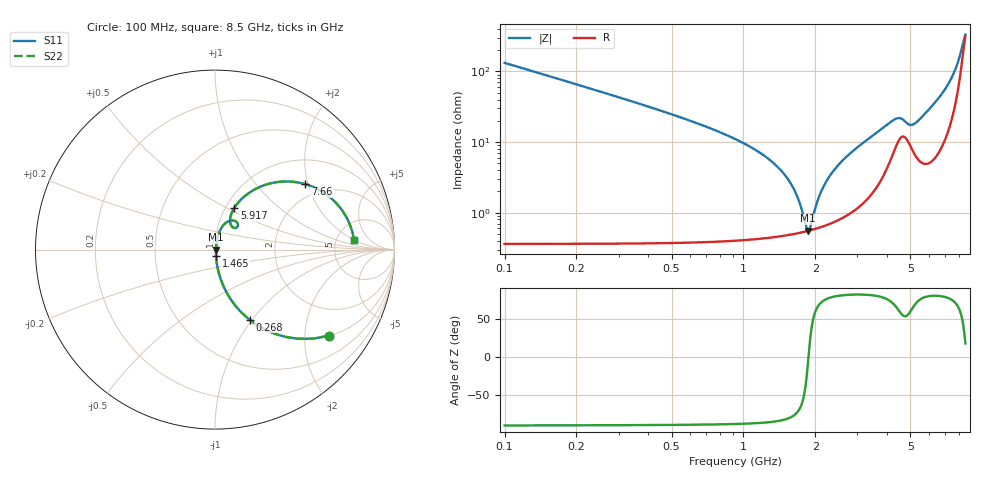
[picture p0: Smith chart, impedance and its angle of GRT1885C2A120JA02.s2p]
!Murata Part Number: GRT1885C2A120JA02
!These Parameters are Measured in Series Mode Connection
!Data Generated on Jun 19, 2026
!  o--ll--o
!Port1  Port2
!  o------o
!Operation Temp=25[degC], DC Bias Voltage=0[V]
!Freq. Start=100[MHz] Stop=9[GHz] 401[Steps]
# Hz S RI R 50
!Freq.(Hz) S11(Real) S11(Imag) S21(Real) S21(Imag) S12(Real) S12(Imag) S22(Real) S22(Imag)
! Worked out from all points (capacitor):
!   401 points, 100 MHz to 8.5 GHz, reference 50 ohm
!   read as one part in series: C = 12 pF near 142 MHz
!   lowest |Z| = 555 mohm at 1.864 GHz (marker M1)
!   series resonance near 1.872 GHz, so ESL is about 600 pH
!   S11 on the Smith chart (normalised r, x): 100 MHz: 1.01, -2.65; 268 MHz: 1.01, -0.97; 1.465 GHz: 1.01, -0.07; 5.917 GHz: 1.10, +0.55; 7.66 GHz: 1.62, +1.92; 8.5 GHz: 7.35, +2.06
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1e8  0.636 -0.4798  0.364 0.4798  0.364 0.4798  0.636 -0.4798
2.05e8  0.2914 -0.4516  0.7086 0.4516  0.7086 0.4516  0.2914 -0.4516
2.68e8  0.1925 -0.3905  0.8075 0.3905  0.8075 0.3905  0.1925 -0.3905
4.15e8  0.0878 -0.277  0.9122 0.277  0.9122 0.277  0.0878 -0.277
6.88e8  0.031 -0.1623  0.969 0.1623  0.969 0.1623  0.031 -0.1623
1.465e9  0.00597 -0.0361  0.994 0.0361  0.994 0.0361  0.00597 -0.0361
1.507e9  0.00576 -0.0319  0.9942 0.0319  0.9942 0.0319  0.00576 -0.0319
1.675e9  0.00532 -0.0164  0.9947 0.0164  0.9947 0.0164  0.00532 -0.0164
1.864e9  0.00548 -0.000648  0.9945 0.000648  0.9945 0.000648  0.00548 -0.000648
1.906e9  0.0056 0.00269  0.9944 -0.00269  0.9944 -0.00269  0.0056 0.00269
2.095e9  0.00644 0.0171  0.9936 -0.0171  0.9936 -0.0171  0.00644 0.0171
2.263e9  0.0076 0.0293  0.9924 -0.0293  0.9924 -0.0293  0.0076 0.0293
2.536e9  0.0104 0.0485  0.9896 -0.0485  0.9896 -0.0485  0.0104 0.0485
2.914e9  0.0163 0.0748  0.9837 -0.0748  0.9837 -0.0748  0.0163 0.0748
4.3e9  0.1018 0.1621  0.8982 -0.1621  0.8982 -0.1621  0.1018 0.1621
5.035e9  0.0952 0.1279  0.9048 -0.1279  0.9048 -0.1279  0.0952 0.1279
5.707e9  0.094 0.2066  0.906 -0.2066  0.906 -0.2066  0.094 0.2066
5.917e9  0.108 0.233  0.892 -0.233  0.892 -0.233  0.108 0.233
7.114e9  0.3102 0.3694  0.6898 -0.3694  0.6898 -0.3694  0.3102 0.3694
7.66e9  0.5034 0.3645  0.4966 -0.3645  0.4966 -0.3645  0.5034 0.3645
8.038e9  0.6574 0.2768  0.3426 -0.2768  0.3426 -0.2768  0.6574 0.2768
8.5e9  0.7742 0.0556  0.2258 -0.0556  0.2258 -0.0556  0.7742 0.0556
